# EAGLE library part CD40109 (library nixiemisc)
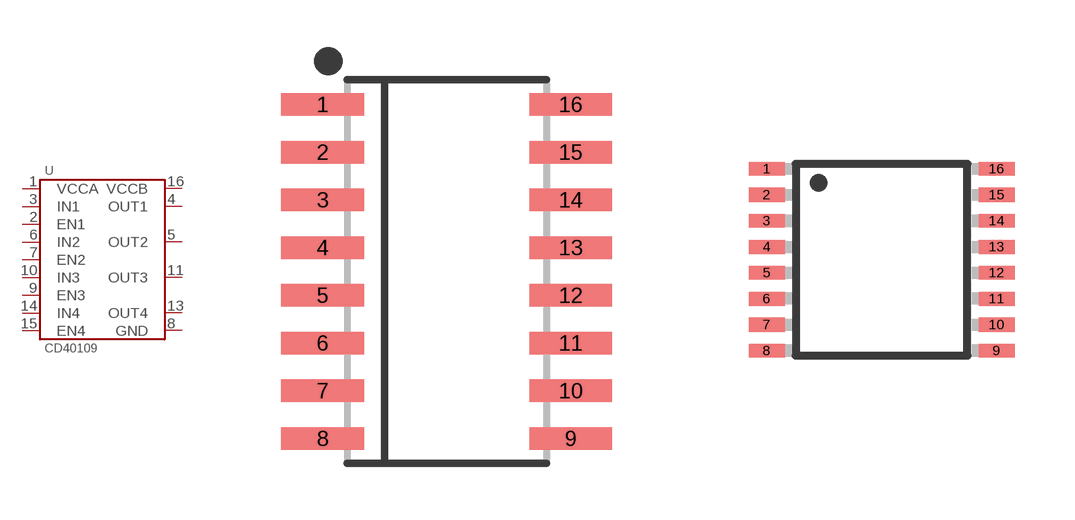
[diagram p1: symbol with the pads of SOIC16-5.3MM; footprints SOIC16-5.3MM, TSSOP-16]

Designator prefix U

## CD40109BNSR  [SOIC16-5.3MM]
1  VCCA
2  EN1
3  IN1
4  OUT1
5  OUT2
6  IN2
7  EN2
8  GND
9  EN3
10  IN3
11  OUT3
13  OUT4
14  IN4
15  EN4
16  VCCB

## CD40109  [TSSOP-16]
Pads as for SOIC16-5.3MM

## CD40109DIP16  [DIP16]
Pads as for SOIC16-5.3MM

## Footprint SOIC16-5.3MM (pad centres in mm)
smd 2.2 x 0.6: 1 -3.3,4.445; 2 -3.3,3.175; 3 -3.3,1.905; 4 -3.3,0.635; 5 -3.3,-0.635; 6 -3.3,-1.905; 7 -3.3,-3.175; 8 -3.3,-4.445; 9 3.3,-4.445; 10 3.3,-3.175; 11 3.3,-1.905; 12 3.3,-0.635; 13 3.3,0.635; 14 3.3,1.905; 15 3.3,3.175; 16 3.3,4.445

## Footprint TSSOP-16 (pad centres in mm)
16-Lead Thin Shrink Small Outline Package [TSSOP] (RU-16) Source: 8x ADG1408_1409.pdf
smd 0.9 x 0.35: 1 -2.875,2.275; 2 -2.875,1.625; 3 -2.875,0.975; 4 -2.875,0.325; 5 -2.875,-0.325; 6 -2.875,-0.975; 7 -2.875,-1.625; 8 -2.875,-2.275; 9 2.875,-2.275; 10 2.875,-1.625; 11 2.875,-0.975; 12 2.875,-0.325; 13 2.875,0.325; 14 2.875,0.975; 15 2.875,1.625; 16 2.875,2.275

## Footprint DIP16 (pad centres in mm)
Dual In Line Package
drill 0.813 pad 1.626: 1 -8.89,-3.81; 2 -6.35,-3.81; 3 -3.81,-3.81; 4 -1.27,-3.81; 5 1.27,-3.81; 6 3.81,-3.81; 7 6.35,-3.81; 8 8.89,-3.81; 9 8.89,3.81; 10 6.35,3.81; 11 3.81,3.81; 12 1.27,3.81; 13 -1.27,3.81; 14 -3.81,3.81; 15 -6.35,3.81; 16 -8.89,3.81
